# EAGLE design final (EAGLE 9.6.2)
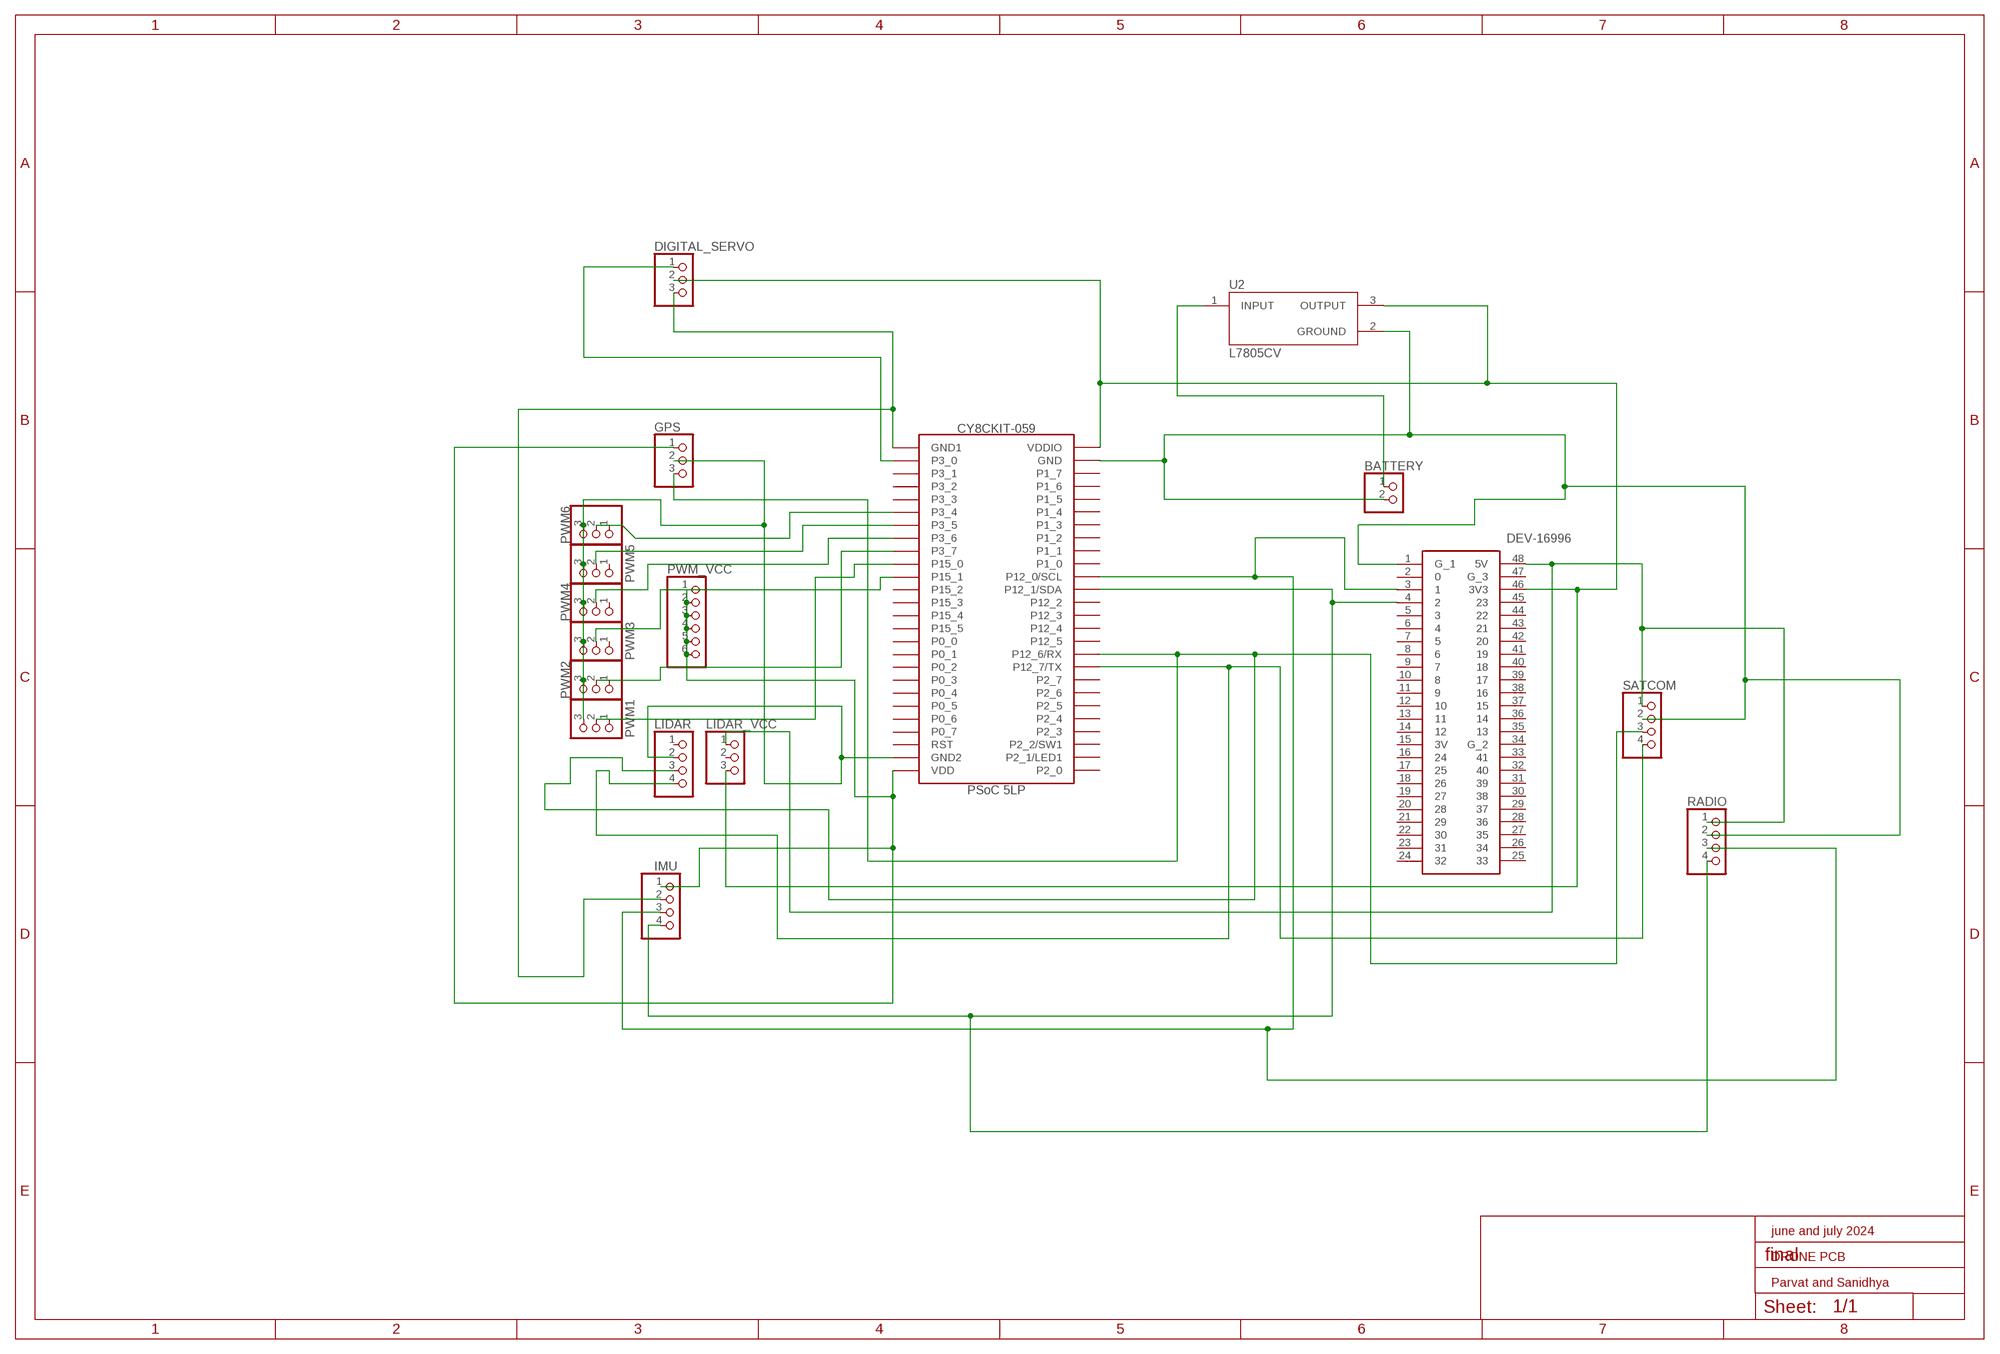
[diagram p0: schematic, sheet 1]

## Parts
BATTERY  PINHD-1X2  [1X02]
DIGITAL_SERVO  PINHD-1X3  [1X03]
DS1  DEV-16996  [DEV16996]
GPS  PINHD-1X3  [1X03]
IMU  PINHD-1X4  [1X04]
LIDAR  PINHD-1X4  [1X04]
LIDAR_VCC  PINHD-1X3  [1X03]
PWM1  PINHD-1X3  [1X03]
PWM2  PINHD-1X3  [1X03]
PWM3  PINHD-1X3  [1X03]
PWM4  PINHD-1X3  [1X03]
PWM5  PINHD-1X3  [1X03]
PWM6  PINHD-1X3  [1X03]
PWM_VCC  PINHD-1X6  [1X06]
RADIO  PINHD-1X4  [1X04]
SATCOM  PINHD-1X4  [1X04]
U1  CY8CKIT-059  [CY8CKIT-059]
U2  L7805CV  [TO255P1040X460X1968-3]

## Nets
N$1: PWM4.2 U1.P3_5(P3_6)
N$3: DIGITAL_SERVO.1 U1.RST(P3_0)
N$4: GPS.1 IMU.1 PWM_VCC.1 PWM_VCC.2 PWM_VCC.3 PWM_VCC.4 PWM_VCC.5 PWM_VCC.6 U1.GND3(VDD)
N$5: GPS.2 LIDAR.2 PWM1.3 PWM2.3 PWM3.3 PWM4.3 PWM5.3 PWM6.3 U1.GND2
N$6: GPS.3 LIDAR.3 SATCOM.3 U1.P12_7(P12_6/RX)
N$7: LIDAR.4 SATCOM.4 U1.P2_7(P12_7/TX)
N$8: BATTERY.2 DS1.1(G_1) RADIO.2 SATCOM.2 U1.P1_7(GND) U2.2(GROUND)
N$9: DS1.3 IMU.3 RADIO.3 U1.P12_1(P12_0/SCL)
N$10: DS1.4 IMU.4 RADIO.4 U1.P12_2(P12_1/SDA)
N$11: PWM3.2 U1.P15_0(P15_1)
N$12: PWM6.1 PWM6.2 U1.P3_3(P3_4)
N$13: PWM5.2 U1.P3_4(P3_5)
N$14: PWM2.1 PWM2.2 U1.P3_6(P3_7)
N$15: PWM1.1 PWM1.2 U1.P3_7(P15_0)
N$16: DS1.48(5V) LIDAR_VCC.1 RADIO.1 SATCOM.1
N$17: DIGITAL_SERVO.3 IMU.2 U1.VDD(GND1)
N$18: DIGITAL_SERVO.2 DS1.46(3V3) LIDAR_VCC.3 U1.VDDIO U2.3(OUTPUT)
N$19: BATTERY.1 U2.1(INPUT)
Unconnected: DS1.2 DS1.5 DS1.6 DS1.7 DS1.8 DS1.9 DS1.10 DS1.11 DS1.12 DS1.13 DS1.14 DS1.15(3V) DS1.16 DS1.17 DS1.18 DS1.19 DS1.20 DS1.21 DS1.22 DS1.23 DS1.24 DS1.25 DS1.26 DS1.27 DS1.28 DS1.29 DS1.30 DS1.31 DS1.32 DS1.33 DS1.34(G_2) DS1.35 DS1.36 DS1.37 DS1.38 DS1.39 DS1.40 DS1.41 DS1.42 DS1.43 DS1.44 DS1.45 DS1.47(G_3) LIDAR.1 LIDAR_VCC.2 PWM3.1 PWM4.1 PWM5.1 U1.GND1(P2_0) U1.P0_0(P0_1) U1.P0_1(P0_2) U1.P0_2(P0_3) U1.P0_3(P0_4) U1.P0_4(P0_5) U1.P0_5(P0_6) U1.P0_6(P0_7) U1.P0_7(RST) U1.P1_0(P1_1) U1.P1_1(P1_2) U1.P1_2(P1_3) U1.P1_3(P1_4) U1.P1_4(P1_5) U1.P1_5(P1_6) U1.P1_6(P1_7) U1.P2_0(P2_1/LED1) U1.P2_1(P2_2/SW1) U1.P2_2(P2_3) U1.P2_3(P2_4) U1.P2_4(P2_5) U1.P2_5(P2_6) U1.P2_6(P2_7) U1.P3_0(P3_1) U1.P3_1(P3_2) U1.P3_2(P3_3) U1.P12_0(P1_0) U1.P12_3(P12_2) U1.P12_4(P12_3) U1.P12_5(P12_4) U1.P12_6(P12_5) U1.P15_1(P15_2) U1.P15_2(P15_3) U1.P15_3(P15_4) U1.P15_4(P15_5) U1.P15_5(P0_0)

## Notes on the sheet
- june and july 2024
- DRONE PCB
- Parvat and Sanidhya

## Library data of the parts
BATTERY = pinhead:PINHD-1X2: PIN HEADER
DIGITAL_SERVO GPS LIDAR_VCC PWM1-PWM6 = pinhead:PINHD-1X3: PIN HEADER
DS1 = DEV-16996:DEV-16996: Development Boards & Kits - ARM ,, Source: Datasheet; ARROW_PART_NUMBER: DEV-16996; ARROW_PRICE-STOCK: https://www.arrow.com/en/products/dev-16996/sparkfun-electronics?region=nac; DESCRIPTION: Development Boards & Kits - ARM ,,; HEIGHT: 4.1mm; MANUFACTURER_NAME: SparkFun; MANUFACTURER_PART_NUMBER: DEV-16996; MOUSER_PART_NUMBER: 474-DEV-16996; MOUSER_PRICE-STOCK: https://www.mouser.co.uk/ProductDetail/SparkFun/DEV-16996?qs=hWgE7mdIu5Su1vq701B2Wg%3D%3D
IMU LIDAR RADIO SATCOM = pinhead:PINHD-1X4: PIN HEADER
PWM_VCC = pinhead:PINHD-1X6: PIN HEADER
U1 = CY8CKIT-059:CY8CKIT-059: Check availability; AVAILABILITY: Not in stock; CHECK_PRICES: https://www.snapeda.com/parts/CY8CKIT059/Cypress+Semiconductor/view-part/?ref=eda; DESCRIPTION: DEV BOARD, PSOC 5 PROTOTYPING; Silicon Manufacturer:Cypress; No. of Bits:32bit; Silicon Family Name:PSoC 5; Core Architecture:ARM; Core Sub-Architecture:Cortex-M3; Silicon Core Number:CY8C5888LTI; Kit Contents:Dev Board CY8C5888LTI, Quick Start Guide; Product Range:-; SVHC:No SVHC (12-Jan-2017); Features:PSoC 5LP CPU, Snap-away Programmer/Debugger, CapSense, PSoC Creator, 3.3V to 5.5V Supply, Micro-USB; MF: Cypress Semiconductor; MP: CY8CKIT059; PACKAGE: None; PRICE: None; SNAPEDA_LINK: https://www.snapeda.com/parts/CY8CKIT059/Cypress+Semiconductor/view-part/?ref=snap
U2 = L7805CV:L7805CV: Standard Regulator Pos 5V 1.5A 3-Pin(3+Tab) TO-220 Standard Regulator Pos 5V 1.5A 3-Pin(3+Tab) TO-220 Check availability; AVAILABILITY: In Stock; CHECK_PRICES: https://www.snapeda.com/parts/L7805C-V/STMicroelectronics/view-part/?ref=eda; DESCRIPTION: Linear Voltage Regulator IC Positive Fixed 1 Output 1.5A TO-220; MF: STMicroelectronics; MP: L7805C-V; PACKAGE: TO-220-3 STMicroelectronics; PRICE: None; PURCHASE-URL: https://www.snapeda.com/api/url_track_click_mouser/?unipart_id=1064554&manufacturer=STMicroelectronics&part_name=L7805C-V&search_term=None; SNAPEDA_LINK: https://www.snapeda.com/parts/L7805C-V/STMicroelectronics/view-part/?ref=snap

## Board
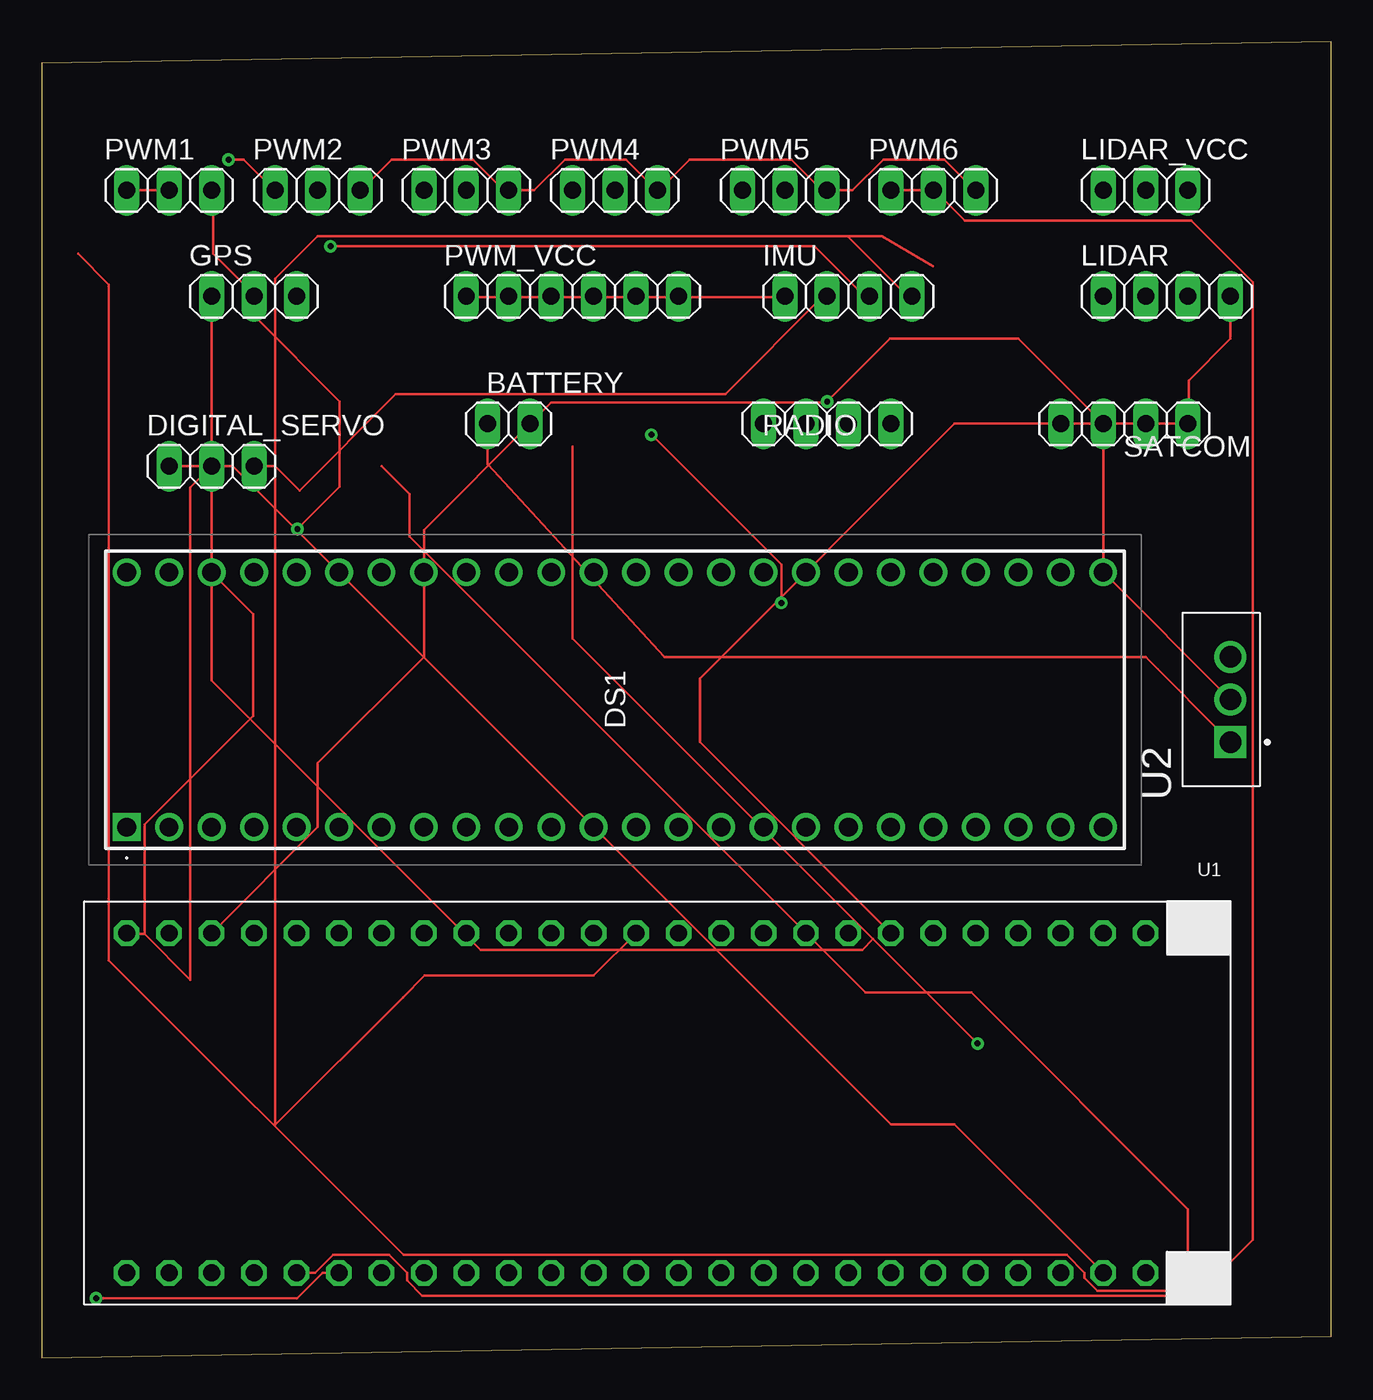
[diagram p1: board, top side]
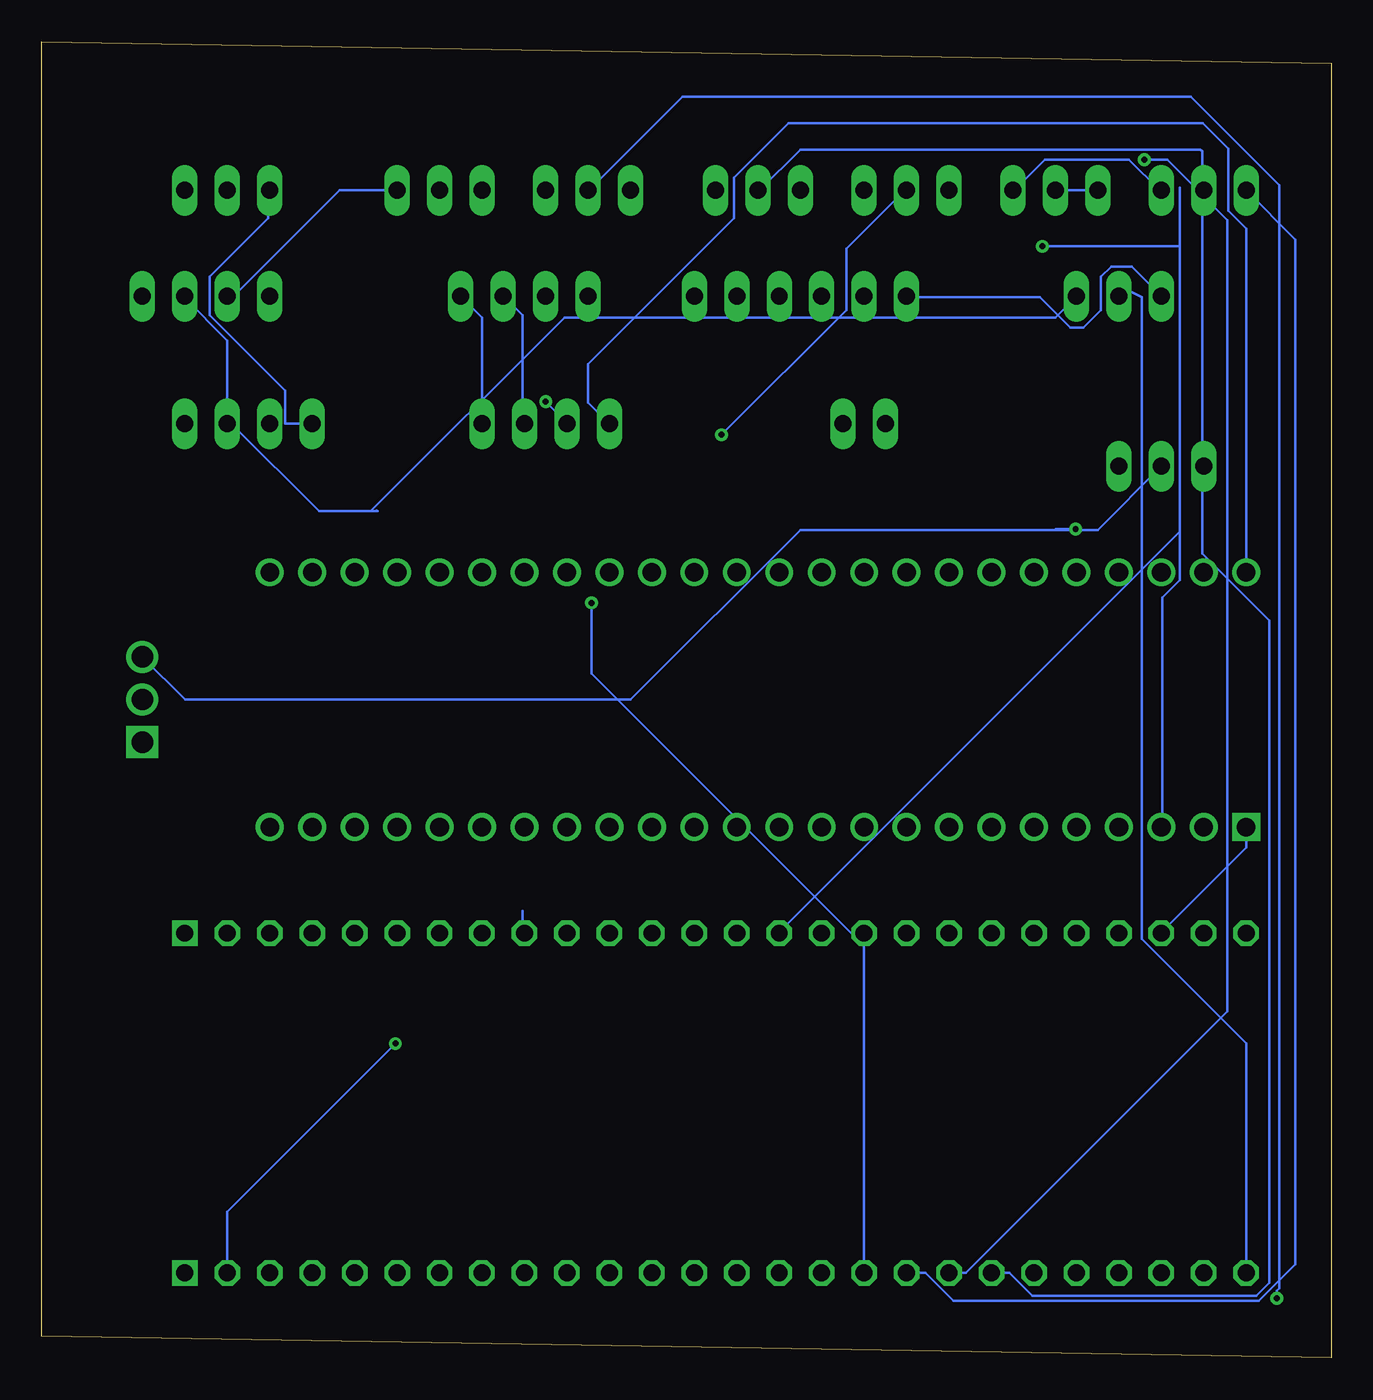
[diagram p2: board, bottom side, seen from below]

Size 77.14 x 78.73 mm. Coordinates in mm from the lower left corner, seen from the top.
Outline: 0,0 77.14,1.27 77.14,78.73 0,77.46 0,0
Copper layers (1*16): Top 0.035mm / dielectric 1.5mm / Bottom 0.035mm
Design rules "default": minimum track width 6mil, minimum drill 0.35mm, track to track 6mil, track to pad 6mil, pad to pad 6mil, via to via 6mil, smd to smd 6mil, copper to edge 40mil, drill to drill 6mil, minimum pad ring 10mil, minimum via ring 8mil, stop-mask expansion 4mil, vias tented up to drill 0mil, thermal gap 10mil

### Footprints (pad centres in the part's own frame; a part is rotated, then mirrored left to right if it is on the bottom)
1X02 = drill 1.016 long: 1 -1.27,0; 2 1.27,0
1X03 = drill 1.016 long: 1 -2.54,0; 2 0,0; 3 2.54,0
DEV16996 = drill 1.11 pad 1.665 square: 1 0,0 | drill 1.11 pad 1.665: 2 0,-2.54; 3 0,-5.08; 4 0,-7.62; 5 0,-10.16; 6 0,-12.7; 7 0,-15.24; 8 0,-17.78; 9 0,-20.32; 10 0,-22.86; 11 0,-25.4; 12 0,-27.94; 13 0,-30.48; 14 0,-33.02; 15 0,-35.56; 16 0,-38.1; 17 0,-40.64; 18 0,-43.18; 19 0,-45.72; 20 0,-48.26; 21 0,-50.8; 22 0,-53.34; 23 0,-55.88; 24 0,-58.42; 25 15.24,-58.42; 26 15.24,-55.88; 27 15.24,-53.34; 28 15.24,-50.8; 29 15.24,-48.26; 30 15.24,-45.72; 31 15.24,-43.18; 32 15.24,-40.64; 33 15.24,-38.1; 34 15.24,-35.56; 35 15.24,-33.02; 36 15.24,-30.48; 37 15.24,-27.94; 38 15.24,-25.4; 39 15.24,-22.86; 40 15.24,-20.32; 41 15.24,-17.78; 42 15.24,-15.24; 43 15.24,-12.7; 44 15.24,-10.16; 45 15.24,-7.62; 46 15.24,-5.08; 47 15.24,-2.54; 48 15.24,0
1X04 = drill 1.016 long: 1 -3.81,0; 2 -1.27,0; 3 1.27,0; 4 3.81,0
1X06 = drill 1.016 long: 1 -6.35,0; 2 -3.81,0; 3 -1.27,0; 4 1.27,0; 5 3.81,0; 6 6.35,0
CY8CKIT-059 = drill 1.016 octagon: GND1 -29.21,10.16; GND2 -31.75,-10.16; GND3 29.21,-10.16; P0_0 6.35,-10.16; P0_1 8.89,-10.16; P0_2 11.43,-10.16; P0_3 13.97,-10.16; P0_4 16.51,-10.16; P0_5 19.05,-10.16; P0_6 21.59,-10.16; P0_7 24.13,-10.16; P1_0 -8.89,10.16; P1_1 -11.43,10.16; P1_2 -13.97,10.16; P1_3 -16.51,10.16; P1_4 -19.05,10.16; P1_5 -21.59,10.16; P1_6 -24.13,10.16; P1_7 -26.67,10.16; P2_1 29.21,10.16; P2_2 26.67,10.16; P2_3 24.13,10.16; P2_4 21.59,10.16; P2_5 19.05,10.16; P2_6 16.51,10.16; P2_7 13.97,10.16; P3_0 -29.21,-10.16; P3_1 -26.67,-10.16; P3_2 -24.13,-10.16; P3_3 -21.59,-10.16; P3_4 -19.05,-10.16; P3_5 -16.51,-10.16; P3_6 -13.97,-10.16; P3_7 -11.43,-10.16; P12_0 -6.35,10.16; P12_1 -3.81,10.16; P12_2 -1.27,10.16; P12_3 1.27,10.16; P12_4 3.81,10.16; P12_5 6.35,10.16; P12_6 8.89,10.16; P12_7 11.43,10.16; P15_0 -8.89,-10.16; P15_1 -6.35,-10.16; P15_2 -3.81,-10.16; P15_3 -1.27,-10.16; P15_4 1.27,-10.16; P15_5 3.81,-10.16; RST 26.67,-10.16; VDDIO -31.75,10.16 | drill 1.016 square: P2_0 31.75,10.16; VDD 31.75,-10.16
TO255P1040X460X1968-3 = drill 1.27 pad 1.91 square: 1 0,0 | drill 1.27 pad 1.91: 2 2.55,0; 3 5.1,0

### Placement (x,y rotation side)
BATTERY  27.94,55.88 0 top
DIGITAL_SERVO  10.16,53.34 0 top
DS1  5.08,31.75 90 top
GPS  12.7,63.5 0 top
IMU  48.26,63.5 0 top
LIDAR  67.31,63.5 0 top
LIDAR_VCC  66.04,69.85 0 top
PWM1  7.62,69.85 0 top
PWM2  16.51,69.85 0 top
PWM3  25.4,69.85 0 top
PWM4  34.29,69.85 0 top
PWM5  44.45,69.85 0 top
PWM6  53.34,69.85 0 top
PWM_VCC  31.75,63.5 0 top
RADIO  46.99,55.88 0 top
SATCOM  64.77,55.88 0 top
U1  36.83,15.24 0 top
U2  71.12,36.83 90 top

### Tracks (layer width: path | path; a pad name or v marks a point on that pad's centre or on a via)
N$1
  Bottom 0.152: U1.P3_5 19.25,5.08 17.88,3.71 4.47,3.71 3.71,4.47 3.71,44.09 7.72,48.11 7.72,72.19 7.82,72.29 31.75,72.29 34.19,69.85 PWM4.2
N$3
  Top 0.152: U1.RST 54.61,13.97 50.8,13.97 11.43,53.34 DIGITAL_SERVO.1
N$4  (via drill 0.35)
  Top 0.152: 49.73,25.04 31.75,43.03 31.75,54.51 | 49.73,25.04 v55.98,18.8 | GPS.1 10.16,40.51 26.26,24.41 49.1,24.41 49.73,25.04 | 27.94,63.45 25.5,63.45 PWM_VCC.1 | 35.56,63.45 33.12,63.45 PWM_VCC.4 32.97,63.45 30.53,63.45 PWM_VCC.3 30.38,63.45 27.94,63.45 | 35.56,63.45 38,63.45 PWM_VCC.6 38.15,63.45 44.4,63.45 IMU.1 | 35.56,63.45 PWM_VCC.5 | 27.94,63.45 PWM_VCC.2
  Bottom 0.152: U1.GND3 66.04,8.74 v55.98,18.8 | GPS.1 11.94,65.28 13.16,65.28 13.77,64.67 13.77,62.69 14.83,61.62 15.6,61.62 17.42,63.45 25.35,63.45 PWM_VCC.1
N$5  (via drill 0.35)
  Top 0.152: v15.29,49.58 17.83,52.12 17.83,57.2 12.7,62.33 GPS.2 12.7,63.6 10.26,66.04 10.26,69.85 PWM1.3 | PWM6.3 55.83,69.85 54,71.68 50.34,71.68 48.51,69.85 PWM5.3 46.69,69.85 44.86,71.68 38.76,71.68 36.93,69.85 PWM4.3 36.78,69.85 34.95,71.68 31.29,71.68 29.46,69.85 PWM3.3 27.63,69.85 25.81,71.68 20.93,71.68 19.1,69.85 PWM2.3
  Bottom 0.152: U1.GND2 5.08,18.8 11.33,25.04 11.33,63.45 12.62,64.09 GPS.2 | v15.29,49.58 16.46,49.58 16.51,49.53 | PWM6.3 59.33,69.85 65.58,63.6 66.04,63.6 LIDAR.2 | PWM2.3 18.95,69.85 17.12,71.68 12.09,71.68 10.26,69.85 PWM1.3
N$6
  Bottom 0.152: 48.36,26.72 48.36,25.5 U1.P12_7 | 57.1,50.7 57.05,50.65 57.46,50.65 | 57.46,50.65 45.87,62.23 16.51,62.23 GPS.3 | LIDAR.3 68.63,63.45 66.04,60.86 SATCOM.3 66.04,55.83 65.73,55.83 60.55,50.65 57.46,50.65
N$7
  Top 0.152: U1.P2_7 39.37,36.83 39.37,40.64 54.61,55.88 SATCOM.4 68.63,55.98 68.63,58.47 71.12,60.96 LIDAR.4
N$8  (via drill 0.35)
  Top 0.152: BATTERY.2 29.21,57.15 | BATTERY.2 22.86,49.53 22.86,41.94 16.51,35.59 16.51,31.75 U1.P1_7 | U2.2 63.51,47 63.5,46.99 SATCOM.2 58.43,60.96 50.75,60.96 v46.99,57.2 46.99,57.15 30.48,57.15 BATTERY.2
  Bottom 0.152: DS1.1 5.08,30.53 10.11,25.5 U1.P1_7 | v46.99,57.2 45.77,55.98 RADIO.2
N$9  (via drill 0.35)
  Top 0.152: v17.27,66.5 46.23,66.5 49.12,63.6 49.43,63.6 IMU.3
  Bottom 0.152: 9.04,49.43 9.04,66.5 | 9.04,66.5 9.04,70 | 9.04,49.43 32.97,25.5 U1.P12_1 | 9.04,49.43 9.04,46.53 10.11,45.47 10.11,31.75 DS1.3 | RADIO.3 48.36,55.98 48.36,62.38 49.43,63.45 IMU.3 | 9.04,66.5 v17.27,66.5
N$10
  Top 0.152: U1.P12_2 33.02,22.86 31.75,22.86 | 31.75,22.86 22.91,22.86 21.61,21.57 13.97,13.92 13.97,64.57 16.51,67.11 48.21,67.11 | 53.31,65.3 50.26,67.11 48.21,67.11 | DS1.4 12.32,31.37 | 48.21,67.11 51.71,63.6 52.02,63.6 IMU.4 | 31.75,22.86
  Bottom 0.152: RADIO.4 50.8,62.23 IMU.4
N$11  (via drill 0.35)
  Top 0.152: v44.25,45.16 44.25,47.45 v36.47,55.22
  Bottom 0.152: U1.P15_0 27.94,24.64 44.25,40.95 v44.25,45.16 | v36.47,55.22 29.01,62.69 29.01,66.34 25.5,69.85 PWM3.2
N$12
  Top 0.152: U1.P3_3 16.36,5.08 17.42,6.15 20.78,6.15 21.84,5.08 21.84,4.62 22.76,3.71 69.09,3.71 72.44,7.06 72.44,64.36 68.78,68.02 55.22,68.02 53.39,69.85 PWM6.2 PWM6.1
N$13  (via drill 0.35)
  Top 0.152: U1.P3_4 16.82,5.08 15.29,3.56 v3.25,3.56
  Bottom 0.152: v3.25,3.56 3.25,4.01 3.1,4.17 3.1,70.16 8.38,75.44 38.81,75.44 44.4,69.85 PWM5.2
N$14  (via drill 0.35)
  Top 0.152: v11.18,71.68 12.09,71.68 13.92,69.85 PWM2.1
  Bottom 0.152: U1.P3_6 21.84,5.08 6.2,20.73 6.2,68.07 9.8,71.68 v11.18,71.68 | PWM2.1 PWM2.2
N$15
  Top 0.152: PWM1.2 PWM1.1
  Bottom 0.152: U1.P3_7 24.28,5.08 22.61,3.4 4.32,3.4 2.13,5.59 2.13,66.9 PWM1.1
N$16
  Bottom 0.152: 43.54,55.27 43.54,55.78 43.49,55.83 43.18,55.83 RADIO.1 44.45,57.15 44.45,59.44 35.71,68.17 35.71,70.61 32.46,73.86 7.67,73.86 6.15,72.34 6.15,68.63 5.08,67.56 DS1.48 | SATCOM.1 62.59,55.88 62.59,57.86 67.11,62.38 67.11,64.67 63.6,68.17 63.6,69.85 LIDAR_VCC.1
N$17
  Top 0.152: 2.18,66.04 4.01,64.21 4.01,23.77 21.64,6.15 61.32,6.15 62.38,5.08 62.38,4.78 63.14,4.01 67.41,4.01 68.48,5.08 U1.VDD 68.58,8.89 55.63,21.84 49.28,21.84 22,49.12 22,51.66 20.32,53.34 | DIGITAL_SERVO.3 13.97,53.34 15.42,51.89 21.18,57.66 40.89,57.66 46.69,63.45 46.99,63.45 IMU.2
N$18
  Top 0.152: 6.15,25.35 5.08,25.35 U1.VDDIO | 6.15,25.35 8.89,22.61 8.89,52.07 DIGITAL_SERVO.2 | DS1.46 12.65,44.5 12.65,38.41 6.15,31.9 6.15,25.35
  Bottom 0.152: DIGITAL_SERVO.2 13.97,49.53 31.75,49.53 41.91,39.37 68.56,39.37 U2.3 | 68.43,69.85 LIDAR_VCC.3 68.63,69.85
N$19
  Top 0.152: U2.1 66.04,41.91 37.25,41.91 26.67,53.46 BATTERY.1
